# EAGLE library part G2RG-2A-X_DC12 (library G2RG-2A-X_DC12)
General Purpose Relays 500VDC/10A high-voltage switching relay (2-pole wiring) Source: Datasheet
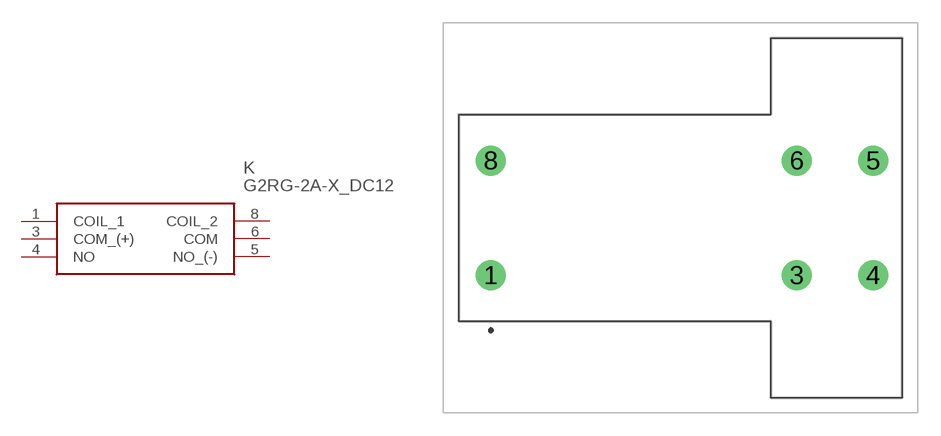
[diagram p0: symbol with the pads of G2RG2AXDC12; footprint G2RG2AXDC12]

Designator prefix K

## G2RG-2A-X_DC12 (Description: General Purpose Relays 500VDC/10A high-voltage switching relay (2-pole wiring); Height: 29.5mm; Manufacturer_Name: Omron Electronics; Manufacturer_Part_Number: G2RG-2A-X DC12)  [G2RG2AXDC12]
1  COIL_1
3  COM_(+)
4  NO
5  NO_(-)
6  COM
8  COIL_2

## Footprint G2RG2AXDC12 (pad centres in mm)
G2RG-2A-X DC12-2
drill 1.3 pad 1.95: 1 0,0; 3 20,0; 4 25,0; 5 25,7.5; 6 20,7.5; 8 0,7.5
